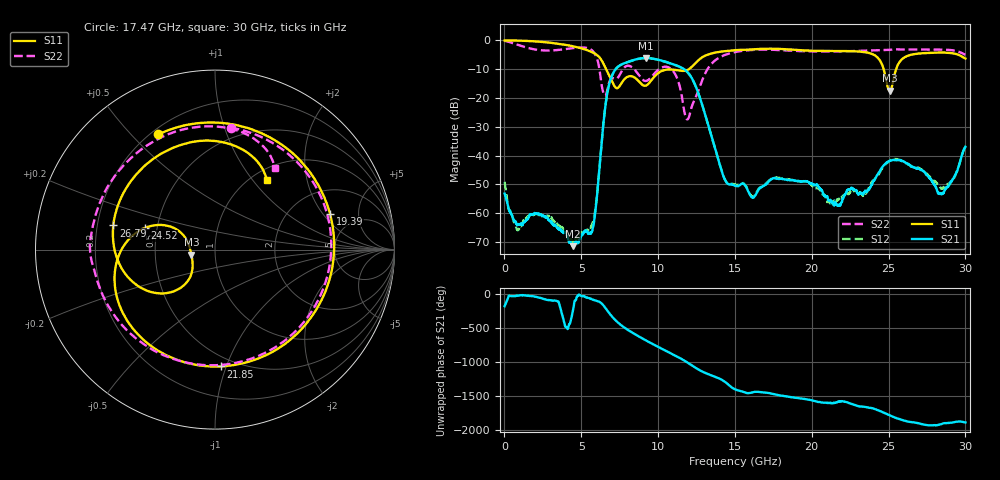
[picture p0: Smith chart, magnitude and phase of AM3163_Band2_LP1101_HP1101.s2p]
!Agilent Technologies,E8364B,MY43040894,A.07.50.67
!Agilent E8364B: A.07.50.67
!Date: Thursday, August 20, 2020 11:14:21
!Correction: S11(Full 2 Port(1,2))
!S21(Full 2 Port(1,2))
!S12(Full 2 Port(1,2))
!S22(Full 2 Port(1,2))
!S2P File: Measurements: S11, S21, S12, S22:
# Hz S  dB  R 50
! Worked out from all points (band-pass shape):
!   3201 points, 10 MHz to 30 GHz, reference 50 ohm
!   highest |S21| = -6.15 dB at 9.204 GHz (marker M1); lowest = -71.4 dB at 4.443 GHz (marker M2)
!   |S21| within 3 dB of the highest: 7.388 GHz to 11.41 GHz (4.017 GHz wide, 42.7 % of centre)
!   lowest |S11| = -17.4 dB at 25.08 GHz (marker M3), VSWR 1.31, Z = 38.3 - j2.21 ohm
!   |S11| at or under -10 dB: 6.614 GHz to 12.01 GHz (5.396 GHz wide, 57.9 % of centre); 24.68 GHz to 25.49 GHz (811.8 MHz wide, 3.24 % of centre)
!   |S22| runs from -27.4 to -0.2 dB; largest |S21 - S12| = 0.0047
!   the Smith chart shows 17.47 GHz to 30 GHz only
!   S11 on the Smith chart (normalised r, x): 17.47 GHz: 0.23, +0.60; 19.39 GHz: 3.24, +2.37; 21.85 GHz: 0.42, -0.96; 24.52 GHz: 0.43, +0.12; 26.79 GHz: 0.27, +0.11; 30 GHz: 1.17, +1.18
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1e7  -0.04 -2.7  -53.19 -178.4  -49.10 -164.0  -0.19 -7.8
8.253531e8  -0.10 -30.6  -63.88 -23.8  -65.83 -30.4  -1.47 -85.4
1.828144e9  -0.31 -68.1  -60.43 -30.8  -60.49 -30.1  -3.02 -171.9
3.130834e9  -0.92 -117.7  -63.70 -97.7  -62.16 81.6  -3.49 92.7
4.442897e9  -2.04 -172.4  -71.44 103.6  -69.84 36.9  -2.70 5.4
5.014581e9  -2.78 159.8  -67.72 -28.7  -66.48 -31.9  -2.47 -33.9
5.801819e9  -4.37 111.4  -64.08 -85.5  -62.07 -110.2  -4.04 -101.2
6.954559e9  -13.60 18.2  -12.85 42.0  -12.90 42.0  -13.29 -81.4
8.201019e9  -12.43 -75.1  -7.18 170.2  -7.23 170.5  -9.01 -120.9
9.203809e9  -15.72 -142.2  -6.15 40.2  -6.16 40.3  -14.11 -135.5
1.000979e10  -11.34 177.3  -6.74 -55.4  -6.77 -55.5  -10.22 -141.7
1.191228e10  -10.30 29.2  -11.03 75.2  -11.14 75.8  -27.42 136.7
1.5005e10  -3.42 -134.7  -50.49 42.4  -49.99 42.9  -4.08 -168.0
1.74698e10  -2.91 116.2  -47.92 -24.7  -47.69 -25.0  -3.28 82.7
1.939104e10  -3.46 17.4  -49.02 -92.1  -48.91 -92.9  -3.78 -0.4
2.000958e10  -3.61 -12.4  -49.77 -118.7  -50.36 -116.3  -3.87 -24.6
2.184647e10  -3.72 -87.1  -57.02 -136.5  -54.47 -132.3  -3.83 -86.8
2.451745e10  -7.74 163.0  -44.52 77.8  -45.00 79.1  -3.41 -158.7
2.500479e10  -17.10 177.6  -41.99 29.2  -42.18 32.2  -3.32 -170.6
2.507977e10  -17.44 -167.8  -41.84 21.8  -41.85 24.1  -3.28 -172.3
2.679482e10  -4.70 166.7  -44.48 -87.3  -44.28 -89.6  -3.19 143.4
3e10  -6.32 53.2  -36.95 -83.2  -36.98 -84.3  -4.99 53.6
